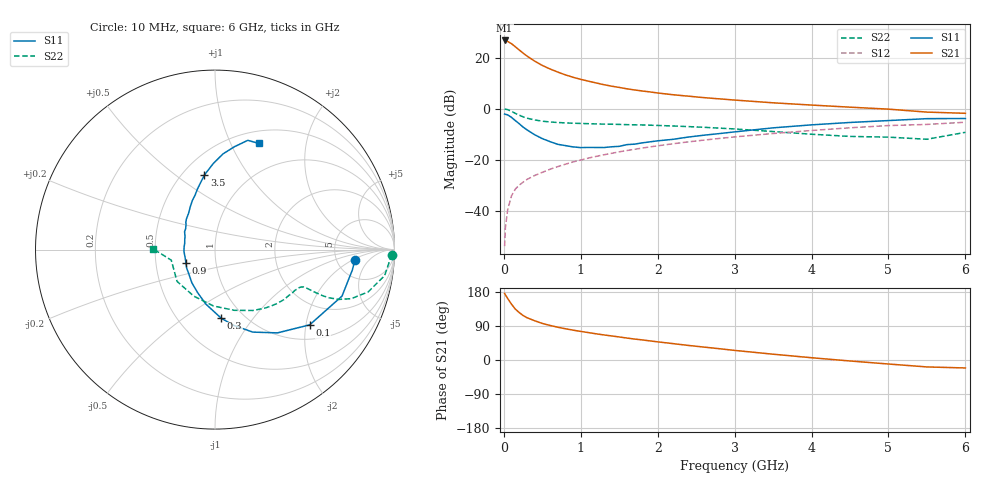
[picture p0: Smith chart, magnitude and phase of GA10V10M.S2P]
! Infineon Technologies  Discrete & RF Semiconductors
! BF775
! Si NPN RF Bipolar Junction Transistor in SOT23
! VCE = 10 V  IC = 10 mA
! Common Emitter S-Parameters:  May  1996
# GHz  S  MA  R  50
!  f  S11  S21  S12  S22
! GHz  MAG  ANG  MAG  ANG  MAG  ANG  MAG  ANG
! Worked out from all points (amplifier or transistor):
!   36 points, 10 MHz to 6 GHz, reference 50 ohm
!   highest |S21| = 26.8 dB at 10 MHz (marker M1)
!   |S21| within 3 dB of that: start of sweep to 170.5 MHz
!   unconditionally stable (mu >= 1): 648.2 MHz to 2.785 GHz
!   at 250 MHz: K = 0.65, MSG = 25.3 dB, |S12| = -28.9 dB
!   at 1.4 GHz: K = 1.09, MAG = 11.3 dB, |S12| = -17.5 dB
!   at 6 GHz: K = 0.88, MSG = 1.8 dB, |S12| = -5.3 dB
!   S11 on the Smith chart (normalised r, x): 10 MHz: 7.51, -2.21; 100 MHz: 1.37, -2.10; 300 MHz: 0.79, -0.71; 900 MHz: 0.71, -0.11; 3.5 GHz: 0.64, +0.64; 6 GHz: 0.64, +1.28
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0.01  0.7819 -4.2  21.77 175.7  0.002 89.3  0.9868 -1.6
0.02  0.7737 -8.4  21.57 172.0  0.0046 83.5  0.9754 -3.6
0.05  0.7537 -20.1  20.8 162.3  0.0104 79.3  0.9562 -8.7
0.1  0.6737 -38.5  18.79 147.1  0.0195 73.0  0.8858 -15.4
0.15  0.5801 -53.1  16.34 134.2  0.0265 66.8  0.8071 -19.8
0.2  0.5056 -65.4  14.17 125.2  0.0316 64.3  0.7442 -21.9
0.25  0.4342 -76.2  12.3 117.5  0.036 62.8  0.6905 -22.9
0.3  0.3839 -84.8  10.79 111.7  0.0408 63.1  0.6504 -23.2
0.4  0.3076 -99.6  8.572 103.6  0.0487 63.3  0.6002 -23.1
0.5  0.2579 -112.2  7.039 96.5  0.0562 64.6  0.5675 -22.9
0.6  0.2253 -124.9  6.004 91.2  0.0646 64.8  0.5476 -22.8
0.7  0.1994 -136.9  5.229 86.5  0.0728 65.9  0.5348 -22.9
0.9  0.1774 -155.9  4.125 78.8  0.09 65.8  0.5174 -24.0
1.1  0.1733 -176.4  3.455 72.3  0.1071 65.8  0.5065 -25.8
1.3  0.1724 168.4  2.952 66.2  0.1242 65.0  0.4971 -27.9
1.6  0.1967 149.5  2.45 57.9  0.1507 63.3  0.4847 -31.7
2.2  0.25 126.1  1.872 43.2  0.2045 59.0  0.4567 -41.3
2.8  0.3237 110.0  1.556 29.8  0.2599 53.5  0.4145 -53.3
3.5  0.4197 98.1  1.301 15.3  0.325 45.9  0.3551 -72.3
4.5  0.5353 85.2  1.068 -2.6  0.421 33.9  0.2849 -114.5
5.5  0.6357 73.3  0.855 -18.3  0.4898 18.8  0.2506 -166.4
6  0.6399 67.6  0.81 -21.0  0.5406 14.7  0.3429 179.5
